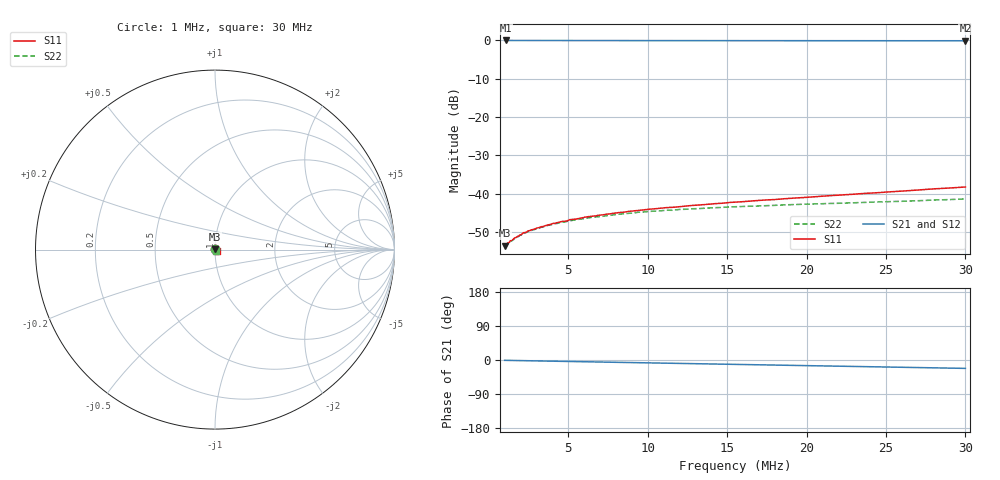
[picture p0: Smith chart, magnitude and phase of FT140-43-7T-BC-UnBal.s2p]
! ListType=Log
!!FT140-43 7TBest Case Balun Unbalanced
# MHZ S RI R 50
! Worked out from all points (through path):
!   101 points, 1 MHz to 30 MHz, reference 50 ohm
!   highest |S21| = -0.01 dB at 1.07 MHz (marker M1); lowest = -0.1 dB at 30 MHz (marker M2)
!   group delay of S21, straight-line fit = 2.04 ns
!   lowest |S11| = -53.6 dB at 1 MHz (marker M3), VSWR 1.00, Z = 50.2 + j0.139 ohm
!   |S11| at or under -10 dB: start of sweep to end of sweep
!   |S22| runs from -53.7 to -41.4 dB; largest |S21 - S12| = 0.00036
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1  0.00157 0.00138  0.9986 -0.0144  0.9987 -0.0144  0.00155 0.00136
1.070391  0.00159 0.00139  0.9986 -0.0153  0.9987 -0.0154  0.00158 0.0014
1.185376  0.00169 0.0015  0.9984 -0.0169  0.9985 -0.0169  0.00166 0.00149
1.226386  0.00169 0.00149  0.9984 -0.0174  0.9985 -0.0174  0.00166 0.00148
1.312713  0.00173 0.00153  0.9983 -0.0186  0.9984 -0.0186  0.00172 0.00157
1.358129  0.00185 0.00157  0.9983 -0.0192  0.9983 -0.0192  0.00178 0.00155
1.723215  0.00207 0.00168  0.9978 -0.0241  0.9979 -0.0241  0.00205 0.00173
1.908328  0.00223 0.00173  0.9977 -0.0265  0.9978 -0.0266  0.00214 0.00176
1.97435  0.00228 0.00178  0.9976 -0.0274  0.9976 -0.0274  0.00222 0.00183
2.042657  0.00228 0.00179  0.9976 -0.0283  0.9976 -0.0283  0.00224 0.00179
2.186442  0.00246 0.00186  0.9974 -0.0302  0.9974 -0.0302  0.00235 0.00183
2.340347  0.00244 0.00192  0.9972 -0.0322  0.9973 -0.0323  0.00245 0.0019
2.505087  0.00262 0.00195  0.9971 -0.0344  0.9971 -0.0344  0.00254 0.00195
4.172448  0.0035 0.00213  0.9951 -0.0561  0.9952 -0.0562  0.00343 0.00214
5.117033  0.004 0.00221  0.9939 -0.0683  0.9939 -0.0684  0.00383 0.00219
5.862773  0.0043 0.00214  0.9929 -0.0778  0.9929 -0.0779  0.00412 0.00217
9.438436  0.00577 0.00178  0.9868 -0.1233  0.9868 -0.1234  0.00541 0.00186
10.81396  0.00626 0.00151  0.984 -0.1406  0.984 -0.1407  0.00574 0.00159
15.72057  0.00778 0.000187  0.9717 -0.2016  0.9717 -0.2018  0.00675 0.000428
20.63659  0.00897 -0.00169  0.9558 -0.2616  0.9558 -0.2619  0.00724 -0.00117
25.30843  0.00978 -0.004  0.9375 -0.3175  0.9374 -0.3178  0.00723 -0.00308
30  0.0101 -0.00675  0.9158 -0.3722  0.9157 -0.3725  0.00671 -0.00524
